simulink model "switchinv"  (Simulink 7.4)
settings: Solver=ode45  StartTime=0.0  StopTime=1/fsw  MaxStep=1e-3  RelTol=1e-3
InitFcn:
  | close all,clear,clc,disp('Pre-loaded frequency and DC voltage'),fsw=50,Vdc=1,To=1/(6*fsw);warning off
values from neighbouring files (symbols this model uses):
  To = 0.02    [fourier0.m]    (also in imdefSIvec1.m = 19.7882645911)
undefined symbols (not defined in the file or in its folder): Vdc
libraries: simulink x2

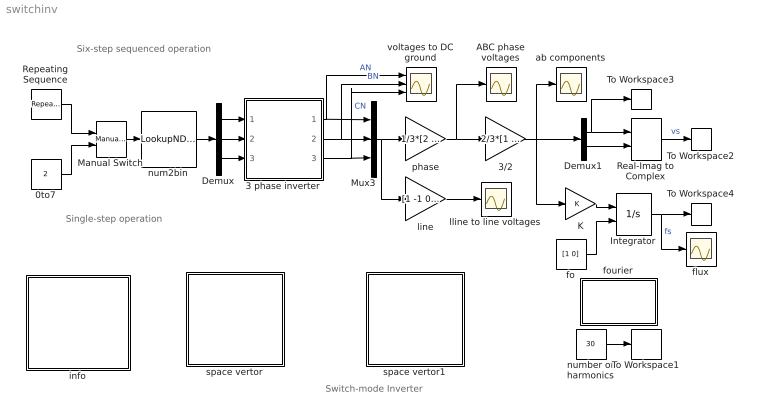
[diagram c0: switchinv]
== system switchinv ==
  note: Switch-mode Inverter
  note: Six-step sequenced operation
  note: Single-step operation
  0to7 : Constant  Value=2  OutDataType=sfix(16)  OutScaling=2^0
  3 phase inverter : Subsystem
  3/2 : Gain  Gain=2/3*[1 -0.5 -0.5;0 sqrt(3)/2 -sqrt(3)/2]  Multiplication=Matrix(K*u)  ParameterDataType=sfix(16)  ParameterScaling=2^0  OutDataType=sfix(16)  OutScaling=2^0
  ABC phase voltages : Scope
  Demux : Demux  Outputs=3
  Demux1 : Demux  Outputs=2
  Integrator : Integrator  InitialConditionSource=external  InitialCondition=[1 0]
  K : Gain  ParameterDataType=sfix(16)  ParameterScaling=2^0  OutDataType=sfix(16)  OutScaling=2^0
  Manual Switch : simulink/Signal Routing/Manual Switch  SystemSampleTime=-1  sw=1  action=0  varsize=off
  Mux3 : Mux  Inputs=3
  Real-Imag to Complex : RealImagToComplex
  Repeating Sequence : simulink/Sources/Repeating Sequence  SystemSampleTime=-1  rep_seq_t="[0 1*To 1*To 2*To  2*To  3*To 3*To 4*To 4*To 5*To 5*To 6*To]"  rep_seq_y="[0 0 1 1 2  2 3  3 4 4 5 5]"
  To Workspace1 : ToWorkspace  VariableName=h  SampleTime=-1  SaveFormat=Array
  To Workspace2 : ToWorkspace  VariableName=vs  SampleTime=-1  SaveFormat=Array
  To Workspace3 : ToWorkspace  VariableName=f  SampleTime=-1  SaveFormat=Array
  To Workspace4 : ToWorkspace  VariableName=fs  SampleTime=-1  SaveFormat=Array
  ab components : Scope
  flux : Scope
  fo : Constant  Value=[1 0]  OutDataType=sfix(16)  OutScaling=2^0
  fourier : Subsystem
  info : Subsystem
  line : Gain  Gain=[1 -1 0;0 1 -1;-1 0 1]  Multiplication=Matrix(K*u)  ParameterDataType=sfix(16)  ParameterScaling=2^0  OutDataType=sfix(16)  OutScaling=2^0
  lline to line voltages : Scope
  num2bin : LookupNDDirect  InputsSelectThisObjectFromTable=Column  Table=[1 0 1;1 0 0;1 1 0;0 1 0;0 1 1;0 0 1;0 0 0;1 1 1]'  ActionForOutOfRangeInput=Error
  number of harmonics : Constant  Value=30  OutDataType=sfix(16)  OutScaling=2^0
  phase : Gain  Gain=1/3*[2 -1 -1;-1 2 -1;-1 -1 2]  Multiplication=Matrix(K*u)  ParameterDataType=sfix(16)  ParameterScaling=2^0  OutDataType=sfix(16)  OutScaling=2^0
  space vertor : Subsystem
  space vertor1 : Subsystem
  voltages to DC ground : Scope  NumInputPorts=3
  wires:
  3/2/1 -> Demux1/1, ab components/1, K/1
  number of harmonics/1 -> To Workspace1/1
  Demux1/2 -> Real-Imag to Complex/2
  Demux1/1 -> Real-Imag to Complex/1, To Workspace3/1
  3 phase inverter/2(vb) -> Mux3/2, voltages to DC ground/2  "BN"
  3 phase inverter/1(va) -> Mux3/1, voltages to DC ground/1  "AN"
  3 phase inverter/3(vc) -> Mux3/3, voltages to DC ground/3  "CN"
  Mux3/1 -> phase/1, line/1
  Real-Imag to Complex/1 -> To Workspace2/1  "vs"
  num2bin/1 -> Demux/1
  Demux/1 -> 3 phase inverter/1(sa)
  Demux/2 -> 3 phase inverter/2(sb)
  Demux/3 -> 3 phase inverter/3(sc)
  phase/1 -> 3/2/1, ABC phase voltages/1
  line/1 -> lline to line voltages/1
  Manual Switch/1 -> num2bin/1
  0to7/1 -> Manual Switch/2
  Repeating Sequence/1 -> Manual Switch/1
  K/1 -> Integrator/1
  Integrator/1 -> To Workspace4/1, flux/1  "fs"
  fo/1 -> Integrator/2

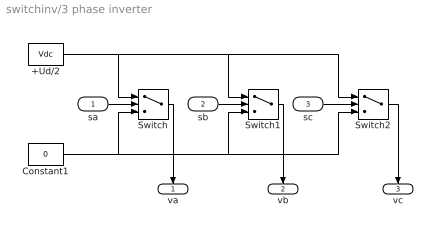
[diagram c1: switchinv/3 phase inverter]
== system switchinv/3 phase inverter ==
  sa : Inport  OutDataType=sfix(16)  OutScaling=2^0
  sb : Inport  Port=2  OutDataType=sfix(16)  OutScaling=2^0
  sc : Inport  Port=3  OutDataType=sfix(16)  OutScaling=2^0
  +Ud/2 : Constant  Value=Vdc  OutDataType=sfix(16)  OutScaling=2^0
  Constant1 : Constant  Value=0  OutDataType=sfix(16)  OutScaling=2^0
  Switch : Switch  Threshold=0.5
  Switch1 : Switch  Threshold=0.5
  Switch2 : Switch  Threshold=0.5
  va : Outport  InitialOutput=0
  vb : Outport  Port=2  InitialOutput=0
  vc : Outport  Port=3  InitialOutput=0
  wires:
  Switch1/1 -> vb/1
  Switch2/1 -> vc/1
  sc/1 -> Switch2/2
  sb/1 -> Switch1/2
  Switch/1 -> va/1
  sa/1 -> Switch/2
  Constant1/1 -> Switch2/3, Switch1/3, Switch/3
  +Ud/2/1 -> Switch2/1, Switch1/1, Switch/1

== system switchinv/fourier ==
  note: To obtain the Fourier decomposition of a periodic signal: a) run a simulation for one period duration b) Specify the fundamental frequency c) Specify the number of harmonics

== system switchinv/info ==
  note: Adjusting the magnitude and frequency of the inverter output
  note: The magnitude and frequency of the 6-step pulse are specified in a callback placed in Model Properties

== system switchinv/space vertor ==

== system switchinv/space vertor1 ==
